TYPE STR_NDO :
STRUCT
	DRY_PUMP_RUN	,
	AV101	,
	AV102	,
	AV103	,
	AV104	,
	AV105	,
	AV106	,
	AV107	,
	AV108	,
	AV109	,	//pin middle
	AV110	,	//pin up
	AV111	,
	AV112	,
	GV101C	,	//门阀打开
	GV101O	,	//门阀关闭
	AV201	,
	AV202	,
	AC101	,
	AC102	,
	AC103	,
	AC104	,
	AC105	,
	AC106	,
	AV1		,
	AV2		,
	AV3		,
	AV4		,
	AV5		,
	AV26	,
	MaualEndStep,
	GV_Open_Enable,
	GV_Close_Enable,
	TM_Robot_Extend_Enable		:BOOL;

END_STRUCT
END_TYPE
